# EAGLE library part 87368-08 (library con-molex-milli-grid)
RECEPTACAL
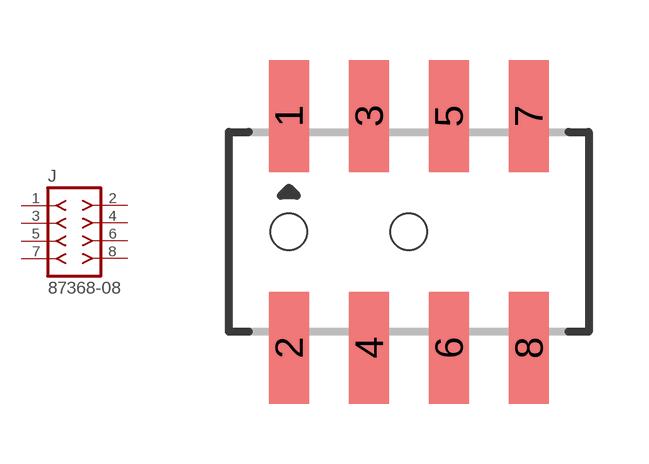
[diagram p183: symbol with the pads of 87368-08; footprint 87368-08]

Designator prefix J

## 87368-08  [87368-08]
1  1  pas
2  2  pas
3  3  pas
4  4  pas
5  5  pas
6  6  pas
7  7  pas
8  8  pas

## Footprint 87368-08 (pad centres in mm)
RECEPTACAL Dual Row, Side Entry
smd 1 x 2.8: 1 -3,2.9; 2 -3,-2.9; 3 -1,2.9; 4 -1,-2.9; 5 1,2.9; 6 1,-2.9; 7 3,2.9; 8 3,-2.9
hole 0.914 at -3,0
hole 0.914 at 0,0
